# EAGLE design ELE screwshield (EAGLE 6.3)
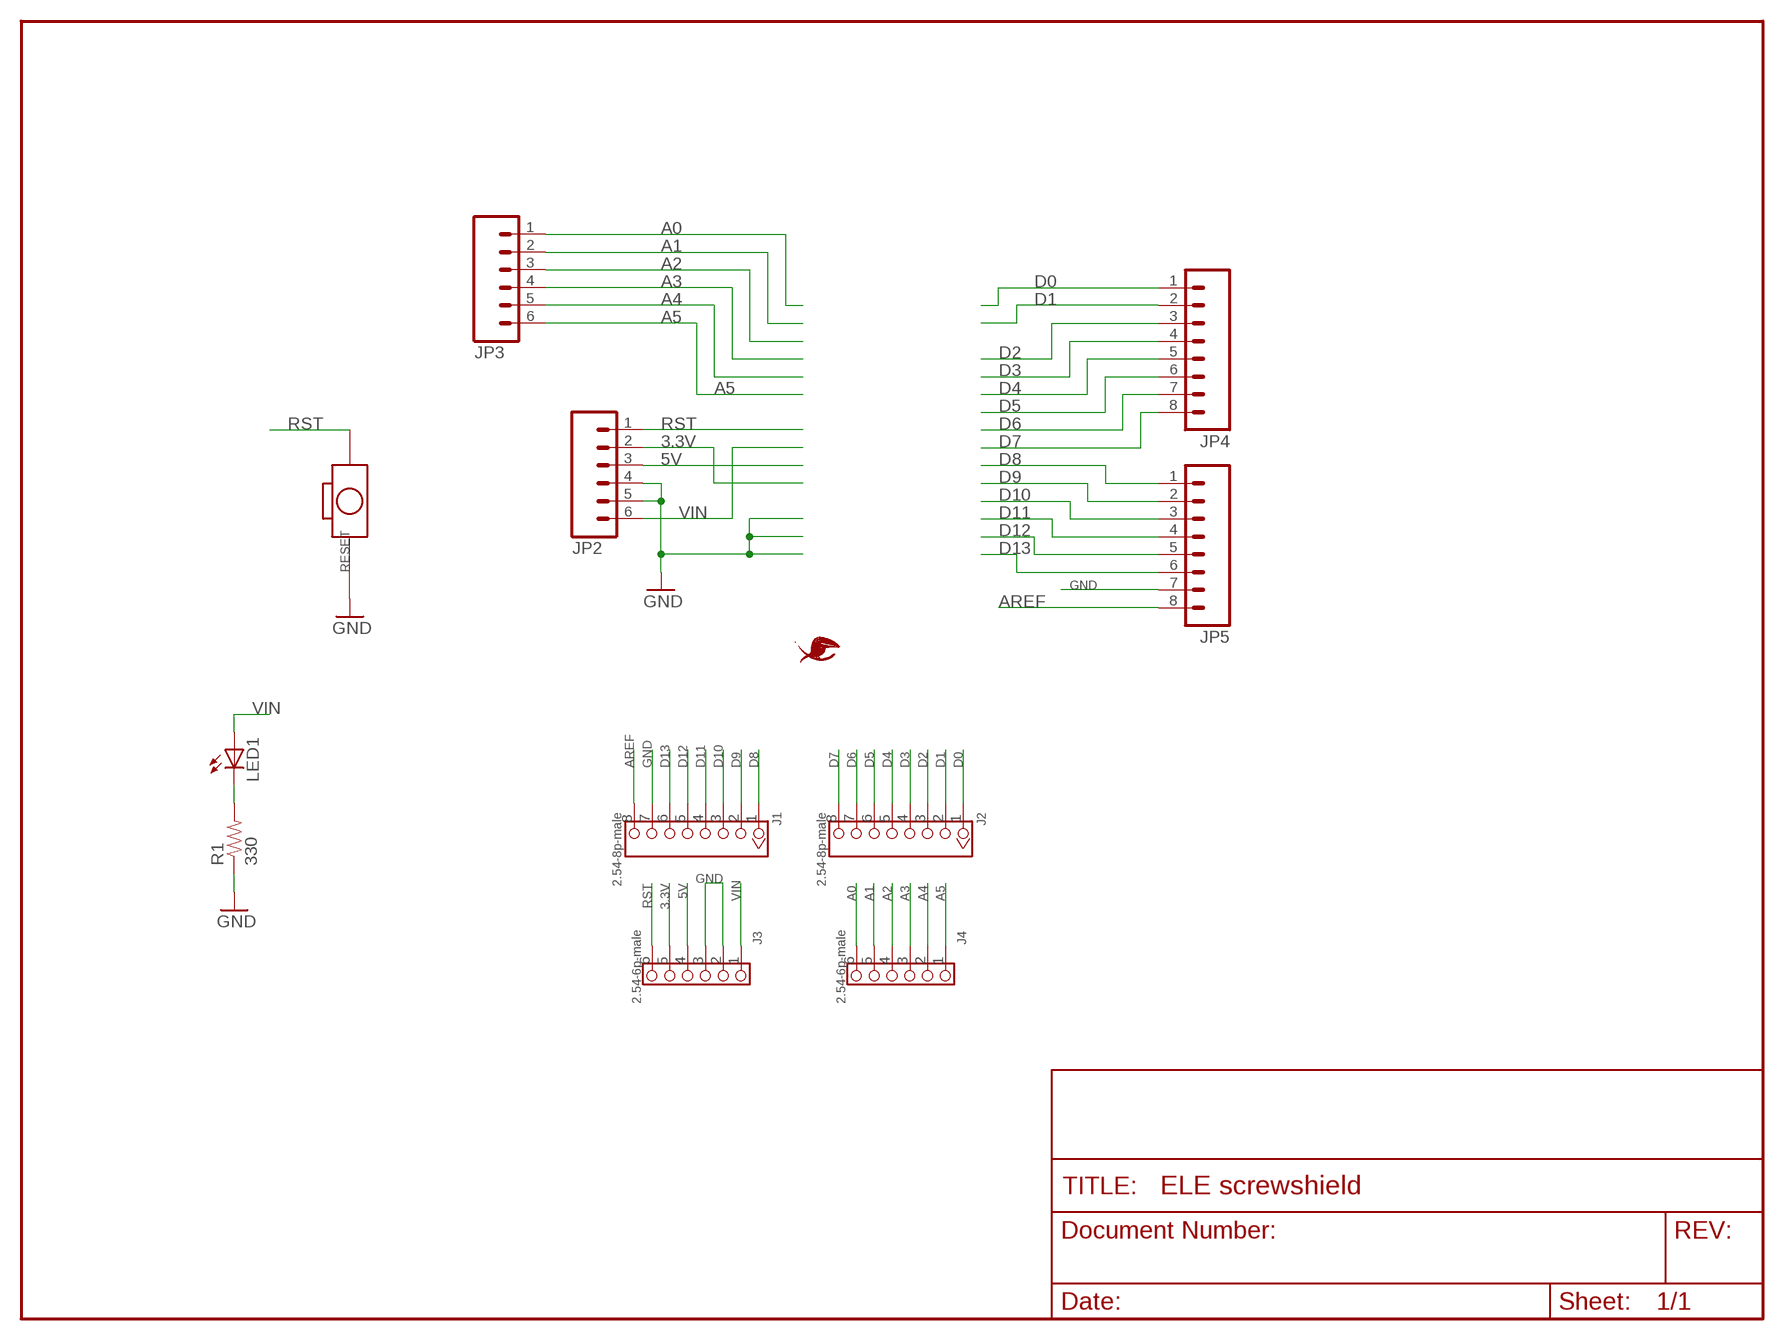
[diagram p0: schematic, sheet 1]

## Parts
J1  2.54-8p-male  HEADER-8P-2.54  [8P-2.54]
J2  2.54-8p-male  HEADER-8P-2.54  [8P-2.54]
J3  2.54-6p-male  HEADER-6P-65/35MIL  [6P-2.54-65/35MIL]
J4  2.54-6p-male  HEADER-6P-65/35MIL  [6P-2.54-65/35MIL]
JP2  M063.5MM-6  [SCREWTERMINAL-3.5MM-6]
JP3  M063.5MM-6  [SCREWTERMINAL-3.5MM-6]
JP4  M083.5MM-8  [SCREWTERMINAL-3.5MM-8]
JP5  M083.5MM-8  [SCREWTERMINAL-3.5MM-8]
LED1  LED5MM  [LED5MM]
R1  330  RESISTORPTH1  [AXIAL-0.3]
RESET  BOTTON-2P-90D  [2P-7.62X3.56-90D]
U$2  ELECROW3  [ELECROW3]

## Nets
3.3V: J3.5 JP2.2
5V: J3.4 JP2.3
A0: J4.6 JP3.1
A1: J4.5 JP3.2
A2: J4.4 JP3.3
A3: J4.3 JP3.4
A4: J4.2 JP3.5
A5: J4.1 JP3.6
AREF: J1.8 JP5.8
D0: J2.1 JP4.1
D1: J2.2 JP4.2
D2: J2.3 JP4.3
D3: J2.4 JP4.4
D4: J2.5 JP4.5
D5: J2.6 JP4.6
D6: J2.7 JP4.7
D7: J2.8 JP4.8
D8: J1.1 JP5.1
D9: J1.2 JP5.2
D10: J1.3 JP5.3
D11: J1.4 JP5.4
D12: J1.5 JP5.5
D13: J1.6 JP5.6
GND: J1.7 J3.2 J3.3 JP2.4 JP2.5 JP5.7 R1.P$1 RESET.P$1
N$6: LED1.K(C) R1.P$2
RST: J3.6 JP2.1 RESET.P$2
VIN: J3.1 JP2.6 LED1.A

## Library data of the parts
J1 J2 = Connector:HEADER-8P
J3 J4 = Connector:HEADER-6P
JP2 JP3 = SparkFun:M06: Header 6 Standard 6-pin 0.1" header. Use with straight break away headers (SKU : PRT-00116), right angle break away headers (PRT-00553), swiss pins (PRT-00743), machine pins (PRT-00117), and female headers (PRT-00115). Molex polarized connector foot print use with SKU : PRT-08094 with associated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
JP4 JP5 = SparkFun:M08: Header 8 Standard 8-pin 0.1" header. Use with straight break away headers (SKU : PRT-00116), right angle break away headers (PRT-00553), swiss pins (PRT-00743), machine pins (PRT-00117), and female headers (PRT-00115).
LED1 = SparkFun:LED: LEDs
R1 = SparkFun:RESISTOR: Resistor
RESET = Discrete:BOTTON-2P
U$2 = ELECROW:ELECROW3

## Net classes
0 default: width 0.152 mm, drill 0.305 mm, clearance 0.152 mm

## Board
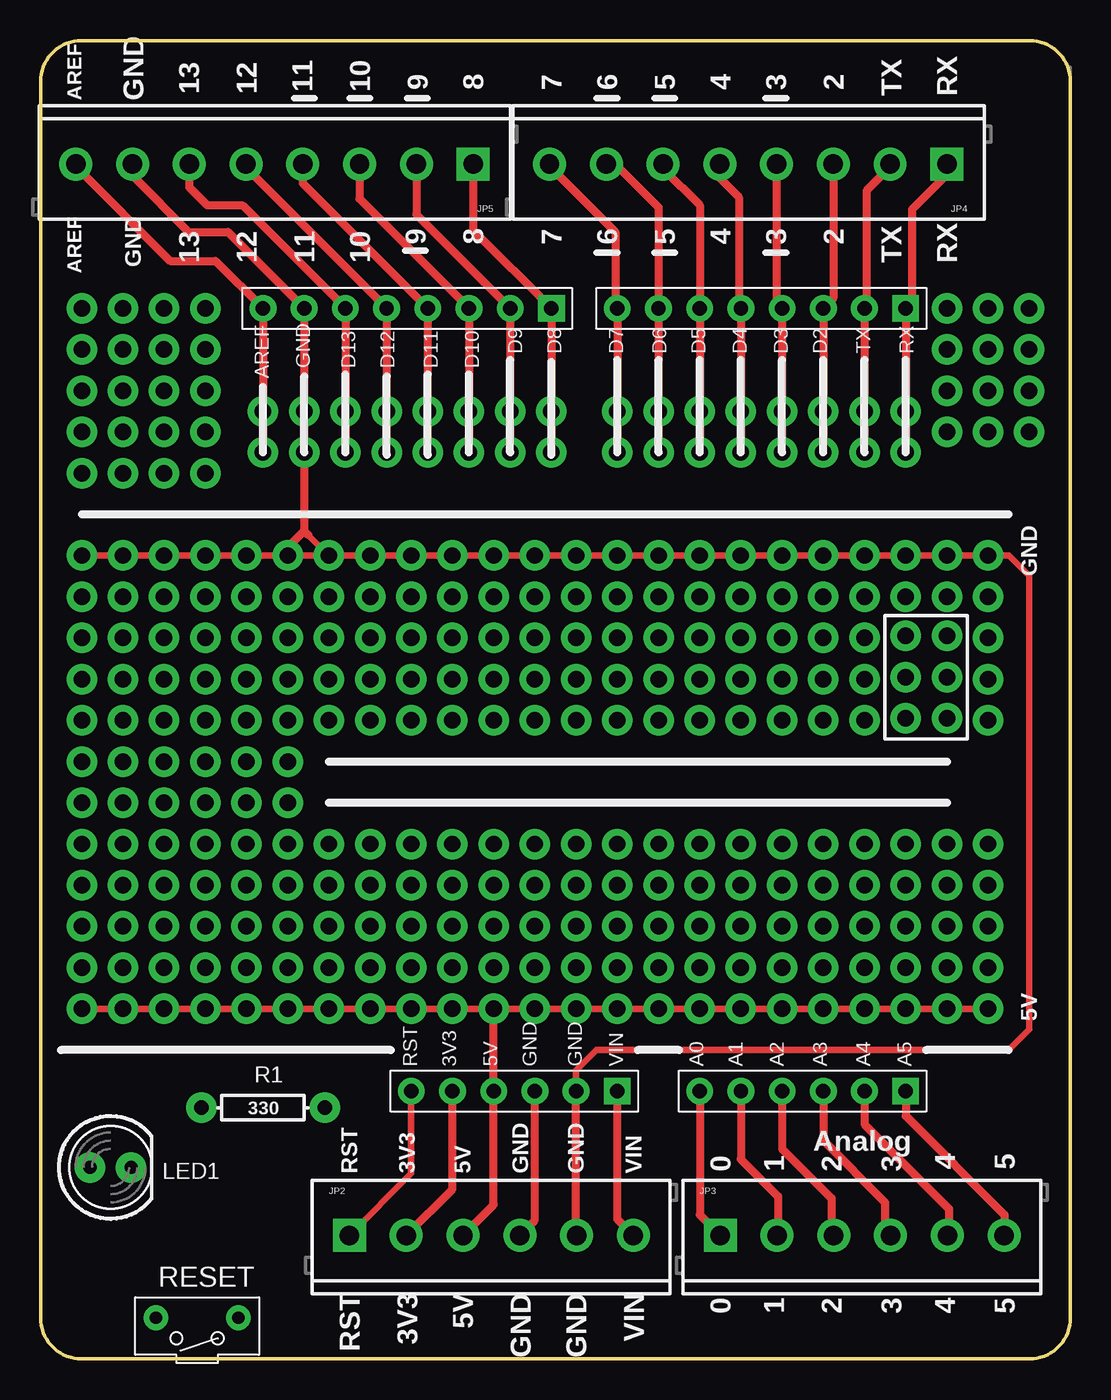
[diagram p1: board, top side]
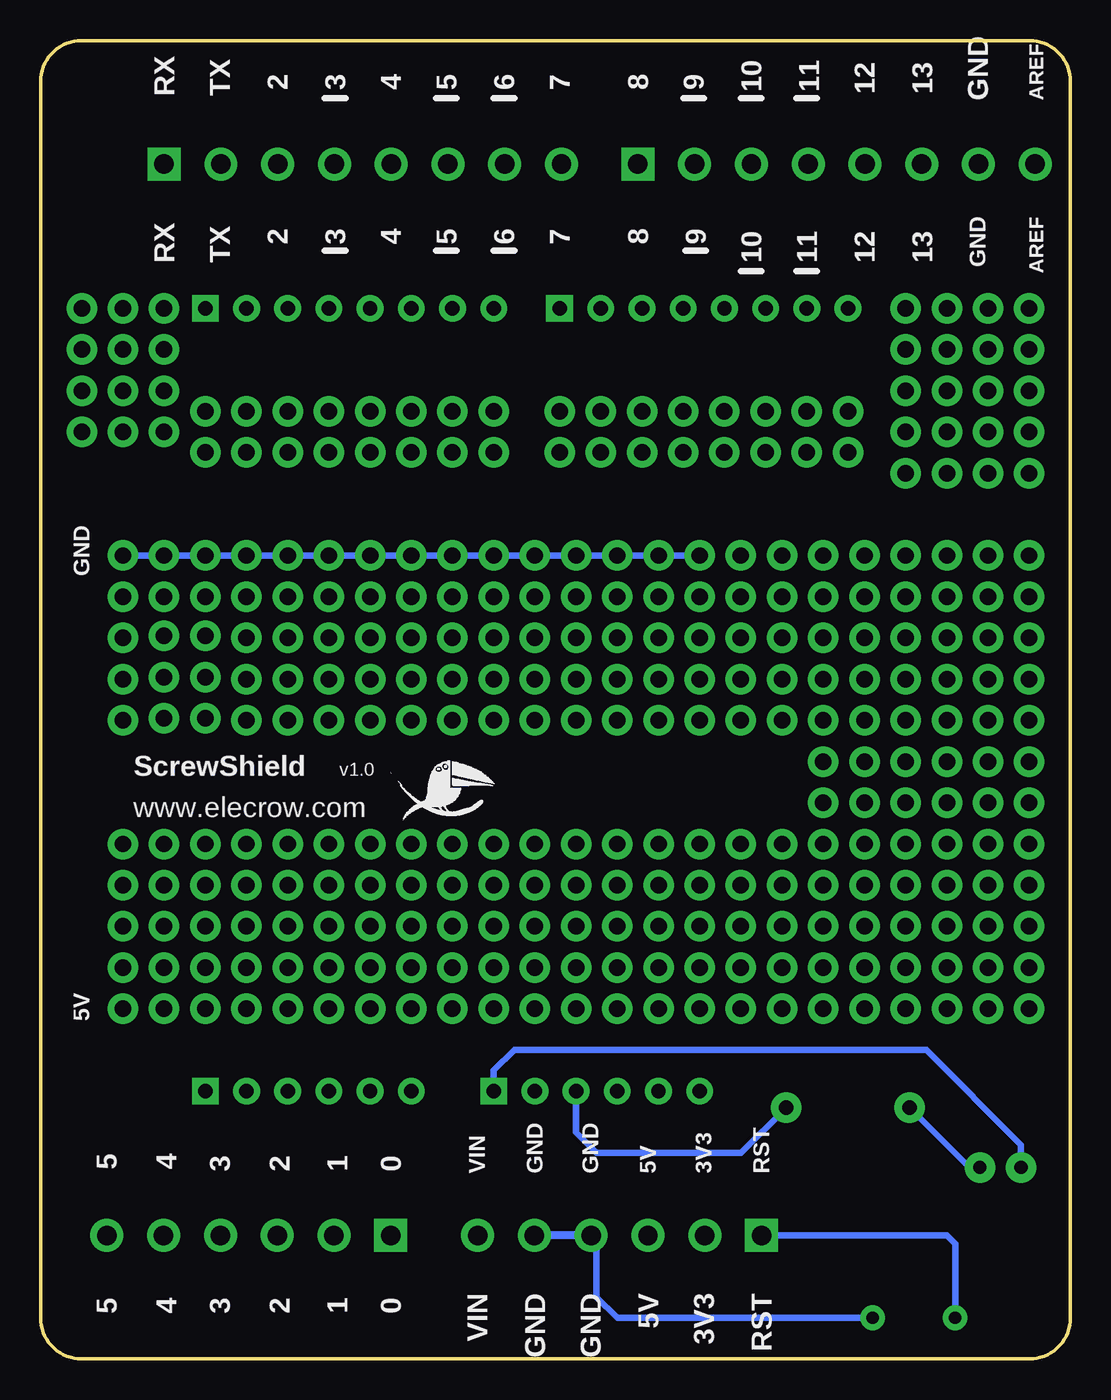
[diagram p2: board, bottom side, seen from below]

Size 63.5 x 81.28 mm. Coordinates in mm from the lower left corner, seen from the top.
Outline: 2.54,0 60.96,0 arc90 63.5,2.54 63.5,78.74 arc90 60.96,81.28 2.54,81.28 arc90 0,78.74 0,2.54 arc90 2.54,0
Copper layers (1*16): Top 0.035mm / dielectric 1.5mm / Bottom 0.035mm
Design rules "SparkFun": minimum track width 8mil, minimum drill 20mil, track to track 8mil, track to pad 8mil, pad to pad 8mil, via to via 8mil, smd to smd 8mil, copper to edge 9mil, drill to drill 8mil, minimum pad ring 12mil, minimum via ring 10mil, stop-mask expansion 4mil, vias tented up to drill 20mil, thermal gap 10mil

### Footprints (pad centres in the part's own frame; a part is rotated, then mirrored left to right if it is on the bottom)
8P-2.54 = drill 0.889 pad 1.651 square: 1 0,8.89 | drill 0.889 pad 1.651: 2 0,6.35; 3 0,3.81; 4 0,1.27; 5 0,-1.27; 6 0,-3.81; 7 0,-6.35; 8 0,-8.89
6P-2.54-65/35MIL = drill 0.889 pad 1.651 square: 1 0,6.35 | drill 0.889 pad 1.651: 2 0,3.81; 3 0,1.27; 4 0,-1.27; 5 0,-3.81; 6 0,-6.35
SCREWTERMINAL-3.5MM-6 = drill 1.2 pad 2.032 square: 1 0,0 | drill 1.2 pad 2.032: 2 3.5,0; 3 7,0; 4 10.5,0; 5 14,0; 6 17.5,0
SCREWTERMINAL-3.5MM-8 = drill 1.2 pad 2.032 square: 1 0,0 | drill 1.2 pad 2.032: 2 3.5,0; 3 7,0; 4 10.5,0; 5 14,0; 6 17.5,0; 7 21,0; 8 24.5,0
LED5MM = drill 0.813 pad 1.88: A -1.27,0; K 1.27,0
AXIAL-0.3 = drill 0.9 pad 1.88: P$1 -3.81,0; P$2 3.81,0
2P-7.62X3.56-90D = drill 0.762 pad 1.524: P$1 0,2.54; P$2 0,-2.54

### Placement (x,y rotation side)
J1  22.61,64.77 270 top
J2  44.45,64.77 270 top
J3  29.21,16.51 270 top
J4  46.99,16.51 270 top
JP2  19.05,7.62 0 top
JP3  41.91,7.62 0 top
JP4  55.88,73.66 180 top
JP5  26.67,73.66 180 top
LED1  4.32,11.81 0 top
R1  13.72,15.49 180 top
RESET  9.65,2.54 270 top
U$2  42.04,32.13 0 bottom

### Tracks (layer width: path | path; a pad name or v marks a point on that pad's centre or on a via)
3.3V
  Top 0.508: J3.5 25.4,10.47 JP2.2
5V  (via drill 1.02 pad 1.88)
  Top 0.406: v2.54,21.59 v5.08,21.59 v7.62,21.59 v10.16,21.59 v12.7,21.59 v15.24,21.59 v17.78,21.59 v20.32,21.59 v22.86,21.59 v25.4,21.59 v27.94,21.59 v30.48,21.59 v33.02,21.59 v35.56,21.59 v38.1,21.59 v40.64,21.59 v43.18,21.59 v45.72,21.59 v48.26,21.59 v50.8,21.59 v53.34,21.59 v55.88,21.59 v58.42,21.59
  Top 0.508: JP2.3 27.94,9.51 J3.4 v27.94,21.59
A0
  Top 0.508: J4.6 40.64,8.89 JP3.1
A1
  Top 0.508: J4.5 43.18,12.32 45.47,10.03 45.47,7.68 JP3.2
A2
  Top 0.508: J4.4 45.72,12.95 48.77,9.91 48.77,7.76 JP3.3
A3
  Top 0.508: J4.3 48.26,13.46 52.07,9.65 52.07,7.96 JP3.4
A4
  Top 0.508: J4.2 50.8,14.48 56.01,9.27 56.01,7.72 JP3.5
A5
  Top 0.508: J4.1 53.34,14.99 59.44,8.89 59.44,7.65 JP3.6
AREF  (via drill 1.02 pad 1.88)
  Top 0.508: JP5.8 2.17,73.52 8,67.69 10.79,67.69 J1.8 v13.72,58.42 v13.72,55.88
D0  (via drill 1.02 pad 1.88)
  Top 0.508: JP4.1 55.88,73.03 53.72,70.87 53.72,65.15 J2.1 v53.34,58.42 v53.34,55.88
D1  (via drill 1.02 pad 1.88)
  Top 0.508: JP4.2 52.38,73.46 50.93,72.01 50.93,64.9 J2.2 v50.8,58.42 v50.8,55.88
D2  (via drill 1.02 pad 1.88)
  Top 0.508: JP4.3 48.88,65.39 J2.3 v48.26,58.42 v48.26,55.88
D3  (via drill 1.02 pad 1.88)
  Top 0.508: JP4.4 45.38,65.11 J2.4 v45.72,58.42 v45.72,55.88
D4  (via drill 1.02 pad 1.88)
  Top 0.508: JP4.5 41.88,72.8 43.05,71.63 43.05,64.9 J2.5 v43.18,58.42 v43.18,55.88
D5  (via drill 1.02 pad 1.88)
  Top 0.508: JP4.6 38.38,73.38 40.64,71.12 J2.6 v40.64,58.42 v40.64,55.88
D6  (via drill 1.02 pad 1.88)
  Top 0.254: 38.1,64.26 J2.7
  Top 0.508: JP4.7 35.43,73.66 38.1,70.99 38.1,64.26 v38.1,58.42 v38.1,55.88
D7  (via drill 1.02 pad 1.88)
  Top 0.508: JP4.8 31.38,73.52 35.43,69.47 35.43,64.9 J2.8 v35.56,58.42 v35.56,55.88
D8  (via drill 1.02 pad 1.88)
  Top 0.508: JP5.1 26.67,69.6 J1.1 v31.5,58.42 v31.5,55.88
D9  (via drill 1.02 pad 1.88)
  Top 0.508: JP5.2 23.17,70.56 J1.2 v28.96,58.42 v28.96,55.88
D10  (via drill 1.02 pad 1.88)
  Top 0.508: JP5.3 19.67,71.52 J1.3 v26.42,58.42 v26.42,55.88
D11  (via drill 1.02 pad 1.88)
  Top 0.508: JP5.4 16.17,72.48 J1.4 v23.88,58.42 v23.88,55.88
D12  (via drill 1.02 pad 1.88)
  Top 0.508: JP5.5 12.67,73.44 J1.5 v21.34,58.42 v21.34,55.88
D13  (via drill 1.02 pad 1.88)
  Top 0.508: JP5.6 9.17,72.24 10.29,71.12 12.45,71.12 J1.6 v18.8,58.42 v18.8,55.88
GND  (via drill 1.02 pad 1.88)
  Top 0.406: J3.2 33.02,17.78 34.29,19.05 59.69,19.05 60.96,20.32 60.96,48.26 59.69,49.53 v58.42,49.53 v20.32,49.53 v17.78,49.53 | v17.78,49.53 v15.24,49.53 v12.7,49.53 v10.16,49.53 v7.62,49.53 v5.08,49.53 v2.54,49.53 | v17.78,49.53 16.51,50.8
  Top 0.508: J3.2 33.02,7.65 JP2.5 | J3.3 30.48,8.55 JP2.4 | JP5.7 5.67,72.94 9.14,69.47 11.56,69.47 J1.7 v16.26,58.42 v16.26,55.88 16.26,51.05 | 16.26,51.05 16.51,50.8 | v15.24,49.53 15.24,50.04 16.26,51.05
  Bottom 0.254: JP2.5 33.02,7.59
  Bottom 0.406: JP2.4 29.21,7.28 29.21,3.81 27.94,2.54 RESET.P$1 | R1.P$1 20.32,12.7 29.21,12.7 30.48,13.97 J3.3 | v22.86,49.53 v25.4,49.53 v27.94,49.53 v30.48,49.53 v33.02,49.53 v35.56,49.53 v38.1,49.53 v40.64,49.53 v43.18,49.53 v45.72,49.53 v48.26,49.53 v50.8,49.53 v53.34,49.53 v55.88,49.53 v58.42,49.53
  Bottom 0.508: JP2.4 JP2.5
N$2  (via drill 1.02 pad 1.88)
  other vias: 25.4,29.21
N$3  (via drill 1.02 pad 1.88)
  other vias: 27.94,29.21
N$4  (via drill 1.02 pad 1.88)
  other vias: 22.86,24.13
N$5  (via drill 1.02 pad 1.88)
  other vias: 10.16,64.77
N$6
  Bottom 0.406: LED1.K 6.22,11.81 R1.P$2
N$9  (via drill 1.02 pad 1.88)
  other vias: 2.54,24.13
N$11  (via drill 1.02 pad 1.88)
  other vias: 5.08,24.13
N$12  (via drill 1.02 pad 1.88)
  other vias: 5.08,59.69
N$13  (via drill 1.02 pad 1.88)
  other vias: 5.08,57.15
N$14  (via drill 1.02 pad 1.88)
  other vias: 7.62,57.15
N$15  (via drill 1.02 pad 1.88)
  other vias: 7.62,59.69
N$16  (via drill 1.02 pad 1.88)
  other vias: 10.16,59.69
N$17  (via drill 1.02 pad 1.88)
  other vias: 10.16,57.15
N$18  (via drill 1.02 pad 1.88)
  other vias: 7.62,24.13
N$19  (via drill 1.02 pad 1.88)
  other vias: 10.16,24.13
N$20  (via drill 1.02 pad 1.88)
  other vias: 12.7,24.13
N$22  (via drill 1.02 pad 1.88)
  other vias: 15.24,24.13
N$24  (via drill 1.02 pad 1.88)
  other vias: 17.78,24.13
N$25  (via drill 1.02 pad 1.88)
  other vias: 20.32,24.13
N$33  (via drill 1.02 pad 1.88)
  other vias: 45.72,24.13
N$34  (via drill 1.02 pad 1.88)
  other vias: 48.26,24.13
N$35  (via drill 1.02 pad 1.88)
  other vias: 50.8,24.13
N$38  (via drill 1.02 pad 1.88)
  other vias: 53.34,24.13
N$39  (via drill 1.02 pad 1.88)
  other vias: 55.88,24.13
N$40  (via drill 1.02 pad 1.88)
  other vias: 58.42,24.13
N$43  (via drill 1.02 pad 1.88)
  other vias: 55.88,59.69
N$44  (via drill 1.02 pad 1.88)
  other vias: 58.42,59.69
N$45  (via drill 1.02 pad 1.88)
  other vias: 60.96,59.69
N$46  (via drill 1.02 pad 1.88)
  other vias: 43.18,24.13
N$49  (via drill 1.02 pad 1.88)
  other vias: 55.88,57.15
N$51  (via drill 1.02 pad 1.88)
  other vias: 58.42,57.15
N$52  (via drill 1.02 pad 1.88)
  other vias: 60.96,57.15
N$53  (via drill 1.02 pad 1.88)
  other vias: 30.48,29.21
N$73  (via drill 1.02 pad 1.88)
  other vias: 33.02,29.21
N$74  (via drill 1.02 pad 1.88)
  other vias: 35.56,29.21
N$75  (via drill 1.02 pad 1.88)
  other vias: 38.1,29.21
N$76  (via drill 1.02 pad 1.88)
  other vias: 40.64,29.21
N$77  (via drill 1.02 pad 1.88)
  other vias: 22.86,29.21
N$78  (via drill 1.02 pad 1.88)
  other vias: 2.54,29.21
N$79  (via drill 1.02 pad 1.88)
  other vias: 2.54,26.67
N$80  (via drill 1.02 pad 1.88)
  other vias: 5.08,29.21
N$81  (via drill 1.02 pad 1.88)
  other vias: 7.62,29.21
N$82  (via drill 1.02 pad 1.88)
  other vias: 10.16,29.21
N$83  (via drill 1.02 pad 1.88)
  other vias: 12.7,29.21
N$84  (via drill 1.02 pad 1.88)
  other vias: 15.24,29.21
N$85  (via drill 1.02 pad 1.88)
  other vias: 17.78,29.21
N$86  (via drill 1.02 pad 1.88)
  other vias: 20.32,29.21
N$87  (via drill 1.02 pad 1.88)
  other vias: 5.08,26.67
N$88  (via drill 1.02 pad 1.88)
  other vias: 7.62,26.67
N$89  (via drill 1.02 pad 1.88)
  other vias: 10.16,26.67
N$90  (via drill 1.02 pad 1.88)
  other vias: 12.7,26.67
N$91  (via drill 1.02 pad 1.88)
  other vias: 15.24,26.67
N$92  (via drill 1.02 pad 1.88)
  other vias: 17.78,26.67
N$93  (via drill 1.02 pad 1.88)
  other vias: 20.32,26.67
N$94  (via drill 1.02 pad 1.88)
  other vias: 25.4,26.67
N$95  (via drill 1.02 pad 1.88)
  other vias: 27.94,26.67
N$96  (via drill 1.02 pad 1.88)
  other vias: 30.48,26.67
N$97  (via drill 1.02 pad 1.88)
  other vias: 33.02,26.67
N$98  (via drill 1.02 pad 1.88)
  other vias: 35.56,26.67
N$99  (via drill 1.02 pad 1.88)
  other vias: 38.1,26.67
N$100  (via drill 1.02 pad 1.88)
  other vias: 40.64,26.67
N$101  (via drill 1.02 pad 1.88)
  other vias: 22.86,26.67
N$102  (via drill 1.02 pad 1.88)
  other vias: 45.72,29.21
N$103  (via drill 1.02 pad 1.88)
  other vias: 48.26,29.21
N$104  (via drill 1.02 pad 1.88)
  other vias: 50.8,29.21
N$105  (via drill 1.02 pad 1.88)
  other vias: 53.34,29.21
N$106  (via drill 1.02 pad 1.88)
  other vias: 55.88,29.21
N$107  (via drill 1.02 pad 1.88)
  other vias: 58.42,29.21
N$108  (via drill 1.02 pad 1.88)
  other vias: 43.18,29.21
N$109  (via drill 1.02 pad 1.88)
  other vias: 2.54,41.91
N$110  (via drill 1.02 pad 1.88)
  other vias: 2.54,39.37
N$111  (via drill 1.02 pad 1.88)
  other vias: 5.08,41.91
N$112  (via drill 1.02 pad 1.88)
  other vias: 7.62,41.91
N$113  (via drill 1.02 pad 1.88)
  other vias: 10.16,41.91
N$114  (via drill 1.02 pad 1.88)
  other vias: 12.7,41.91
N$115  (via drill 1.02 pad 1.88)
  other vias: 15.24,41.91
N$116  (via drill 1.02 pad 1.88)
  other vias: 5.08,39.37
N$117  (via drill 1.02 pad 1.88)
  other vias: 7.62,39.37
N$118  (via drill 1.02 pad 1.88)
  other vias: 10.16,39.37
N$119  (via drill 1.02 pad 1.88)
  other vias: 12.7,39.37
N$120  (via drill 1.02 pad 1.88)
  other vias: 15.24,39.37
N$121  (via drill 1.02 pad 1.88)
  other vias: 2.54,46.99
N$122  (via drill 1.02 pad 1.88)
  other vias: 2.54,44.45
N$123  (via drill 1.02 pad 1.88)
  other vias: 5.08,46.99
N$124  (via drill 1.02 pad 1.88)
  other vias: 7.62,46.99
N$125  (via drill 1.02 pad 1.88)
  other vias: 10.16,46.99
N$126  (via drill 1.02 pad 1.88)
  other vias: 12.7,46.99
N$127  (via drill 1.02 pad 1.88)
  other vias: 15.24,46.99
N$128  (via drill 1.02 pad 1.88)
  other vias: 5.08,44.45
N$129  (via drill 1.02 pad 1.88)
  other vias: 45.72,26.67
N$130  (via drill 1.02 pad 1.88)
  other vias: 7.62,44.45
N$131  (via drill 1.02 pad 1.88)
  other vias: 10.16,44.45
N$132  (via drill 1.02 pad 1.88)
  other vias: 12.7,44.45
N$133  (via drill 1.02 pad 1.88)
  other vias: 15.24,44.45
N$140  (via drill 1.02 pad 1.88)
  other vias: 2.54,36.83
N$141  (via drill 1.02 pad 1.88)
  other vias: 2.54,34.29
N$142  (via drill 1.02 pad 1.88)
  other vias: 5.08,36.83
N$143  (via drill 1.02 pad 1.88)
  other vias: 7.62,36.83
N$144  (via drill 1.02 pad 1.88)
  other vias: 10.16,36.83
N$145  (via drill 1.02 pad 1.88)
  other vias: 12.7,36.83
N$146  (via drill 1.02 pad 1.88)
  other vias: 15.24,36.83
N$147  (via drill 1.02 pad 1.88)
  other vias: 5.08,34.29
N$148  (via drill 1.02 pad 1.88)
  other vias: 7.62,34.29
N$149  (via drill 1.02 pad 1.88)
  other vias: 10.16,34.29
N$150  (via drill 1.02 pad 1.88)
  other vias: 48.26,26.67
N$151  (via drill 1.02 pad 1.88)
  other vias: 50.8,26.67
N$152  (via drill 1.02 pad 1.88)
  other vias: 53.34,26.67
N$153  (via drill 1.02 pad 1.88)
  other vias: 55.88,26.67
N$154  (via drill 1.02 pad 1.88)
  other vias: 58.42,26.67
N$155  (via drill 1.02 pad 1.88)
  other vias: 43.18,26.67
N$156  (via drill 1.02 pad 1.88)
  other vias: 25.4,31.75
N$157  (via drill 1.02 pad 1.88)
  other vias: 27.94,31.75
N$158  (via drill 1.02 pad 1.88)
  other vias: 30.48,31.75
N$159  (via drill 1.02 pad 1.88)
  other vias: 33.02,31.75
N$160  (via drill 1.02 pad 1.88)
  other vias: 35.56,31.75
N$161  (via drill 1.02 pad 1.88)
  other vias: 38.1,31.75
N$162  (via drill 1.02 pad 1.88)
  other vias: 40.64,31.75
N$163  (via drill 1.02 pad 1.88)
  other vias: 22.86,31.75
N$164  (via drill 1.02 pad 1.88)
  other vias: 2.54,31.75
N$165  (via drill 1.02 pad 1.88)
  other vias: 5.08,31.75
N$166  (via drill 1.02 pad 1.88)
  other vias: 7.62,31.75
N$167  (via drill 1.02 pad 1.88)
  other vias: 10.16,31.75
N$168  (via drill 1.02 pad 1.88)
  other vias: 12.7,31.75
N$169  (via drill 1.02 pad 1.88)
  other vias: 15.24,31.75
N$170  (via drill 1.02 pad 1.88)
  other vias: 17.78,31.75
N$171  (via drill 1.02 pad 1.88)
  other vias: 20.32,31.75
N$172  (via drill 1.02 pad 1.88)
  other vias: 45.72,31.75
N$173  (via drill 1.02 pad 1.88)
  other vias: 48.26,31.75
N$174  (via drill 1.02 pad 1.88)
  other vias: 50.8,31.75
N$175  (via drill 1.02 pad 1.88)
  other vias: 53.34,31.75
N$176  (via drill 1.02 pad 1.88)
  other vias: 55.88,31.75
N$177  (via drill 1.02 pad 1.88)
  other vias: 58.42,31.75
N$178  (via drill 1.02 pad 1.88)
  other vias: 43.18,31.75
N$179  (via drill 1.02 pad 1.88)
  other vias: 12.7,34.29
N$180  (via drill 1.02 pad 1.88)
  other vias: 15.24,34.29
N$194  (via drill 1.02 pad 1.88)
  other vias: 17.78,39.37
N$195  (via drill 1.02 pad 1.88)
  other vias: 20.32,39.37
N$196  (via drill 1.02 pad 1.88)
  other vias: 22.86,39.37
N$197  (via drill 1.02 pad 1.88)
  other vias: 25.4,39.37
N$198  (via drill 1.02 pad 1.88)
  other vias: 27.94,39.37
N$199  (via drill 1.02 pad 1.88)
  other vias: 30.48,39.37
N$200  (via drill 1.02 pad 1.88)
  other vias: 33.02,39.37
N$201  (via drill 1.02 pad 1.88)
  other vias: 35.56,39.37
N$202  (via drill 1.02 pad 1.88)
  other vias: 38.1,39.37
N$203  (via drill 1.02 pad 1.88)
  other vias: 40.64,39.37
N$204  (via drill 1.02 pad 1.88)
  other vias: 43.18,39.37
N$205  (via drill 1.02 pad 1.88)
  other vias: 45.72,39.37
N$206  (via drill 1.02 pad 1.88)
  other vias: 48.26,39.37
N$207  (via drill 1.02 pad 1.88)
  other vias: 50.8,39.37
N$208  (via drill 1.02 pad 1.88)
  other vias: 53.34,39.5
N$209  (via drill 1.02 pad 1.88)
  other vias: 55.88,39.5
N$210  (via drill 1.02 pad 1.88)
  other vias: 58.42,39.37
N$221  (via drill 1.02 pad 1.88)
  other vias: 17.78,41.91
N$222  (via drill 1.02 pad 1.88)
  other vias: 20.32,41.91
N$223  (via drill 1.02 pad 1.88)
  other vias: 22.86,41.91
N$224  (via drill 1.02 pad 1.88)
  other vias: 25.4,41.91
N$225  (via drill 1.02 pad 1.88)
  other vias: 27.94,41.91
N$226  (via drill 1.02 pad 1.88)
  other vias: 30.48,41.91
N$227  (via drill 1.02 pad 1.88)
  other vias: 33.02,41.91
N$228  (via drill 1.02 pad 1.88)
  other vias: 35.56,41.91
N$229  (via drill 1.02 pad 1.88)
  other vias: 38.1,41.91
N$230  (via drill 1.02 pad 1.88)
  other vias: 40.64,41.91
N$231  (via drill 1.02 pad 1.88)
  other vias: 43.18,41.91
N$232  (via drill 1.02 pad 1.88)
  other vias: 45.72,41.91
N$233  (via drill 1.02 pad 1.88)
  other vias: 48.26,41.91
N$234  (via drill 1.02 pad 1.88)
  other vias: 50.8,41.91
N$235  (via drill 1.02 pad 1.88)
  other vias: 53.34,42.04
N$236  (via drill 1.02 pad 1.88)
  other vias: 55.88,42.04
N$237  (via drill 1.02 pad 1.88)
  other vias: 58.42,41.91
N$248  (via drill 1.02 pad 1.88)
  other vias: 17.78,44.45
N$249  (via drill 1.02 pad 1.88)
  other vias: 20.32,44.45
N$250  (via drill 1.02 pad 1.88)
  other vias: 22.86,44.45
N$251  (via drill 1.02 pad 1.88)
  other vias: 25.4,44.45
N$252  (via drill 1.02 pad 1.88)
  other vias: 27.94,44.45
N$253  (via drill 1.02 pad 1.88)
  other vias: 30.48,44.45
N$254  (via drill 1.02 pad 1.88)
  other vias: 33.02,44.45
N$255  (via drill 1.02 pad 1.88)
  other vias: 35.56,44.45
N$256  (via drill 1.02 pad 1.88)
  other vias: 38.1,44.45
N$257  (via drill 1.02 pad 1.88)
  other vias: 40.64,44.45
N$258  (via drill 1.02 pad 1.88)
  other vias: 43.18,44.45
N$259  (via drill 1.02 pad 1.88)
  other vias: 45.72,44.45
N$260  (via drill 1.02 pad 1.88)
  other vias: 48.26,44.45
N$261  (via drill 1.02 pad 1.88)
  other vias: 50.8,44.45
N$262  (via drill 1.02 pad 1.88)
  other vias: 53.34,44.58
N$263  (via drill 1.02 pad 1.88)
  other vias: 55.88,44.58
N$264  (via drill 1.02 pad 1.88)
  other vias: 58.42,44.45
N$275  (via drill 1.02 pad 1.88)
  other vias: 17.78,46.99
N$276  (via drill 1.02 pad 1.88)
  other vias: 20.32,46.99
N$277  (via drill 1.02 pad 1.88)
  other vias: 22.86,46.99
N$278  (via drill 1.02 pad 1.88)
  other vias: 25.4,46.99
N$279  (via drill 1.02 pad 1.88)
  other vias: 27.94,46.99
N$280  (via drill 1.02 pad 1.88)
  other vias: 30.48,46.99
N$281  (via drill 1.02 pad 1.88)
  other vias: 33.02,46.99
N$282  (via drill 1.02 pad 1.88)
  other vias: 35.56,46.99
N$283  (via drill 1.02 pad 1.88)
  other vias: 38.1,46.99
N$284  (via drill 1.02 pad 1.88)
  other vias: 40.64,46.99
N$285  (via drill 1.02 pad 1.88)
  other vias: 43.18,46.99
N$286  (via drill 1.02 pad 1.88)
  other vias: 45.72,46.99
N$287  (via drill 1.02 pad 1.88)
  other vias: 48.26,46.99
N$288  (via drill 1.02 pad 1.88)
  other vias: 50.8,46.99
N$289  (via drill 1.02 pad 1.88)
  other vias: 53.34,46.99
N$290  (via drill 1.02 pad 1.88)
  other vias: 55.88,46.99
N$291  (via drill 1.02 pad 1.88)
  other vias: 58.42,46.99
N$350  (via drill 1.02 pad 1.88)
  other vias: 2.54,54.61
N$351  (via drill 1.02 pad 1.88)
  other vias: 5.08,54.61
N$352  (via drill 1.02 pad 1.88)
  other vias: 7.62,54.61
N$353  (via drill 1.02 pad 1.88)
  other vias: 10.16,54.61
N$377  (via drill 1.02 pad 1.88)
  other vias: 2.54,57.15
N$404  (via drill 1.02 pad 1.88)
  other vias: 2.54,59.69
N$439  (via drill 1.02 pad 1.88)
  other vias: 25.4,24.13
N$440  (via drill 1.02 pad 1.88)
  other vias: 27.94,24.13
N$441  (via drill 1.02 pad 1.88)
  other vias: 30.48,24.13
N$442  (via drill 1.02 pad 1.88)
  other vias: 33.02,24.13
N$443  (via drill 1.02 pad 1.88)
  other vias: 35.56,24.13
N$444  (via drill 1.02 pad 1.88)
  other vias: 38.1,24.13
N$445  (via drill 1.02 pad 1.88)
  other vias: 40.64,24.13
N$447  (via drill 1.02 pad 1.88)
  other vias: 2.54,62.23
N$448  (via drill 1.02 pad 1.88)
  other vias: 5.08,62.23
N$449  (via drill 1.02 pad 1.88)
  other vias: 7.62,62.23
N$455  (via drill 1.02 pad 1.88)
  other vias: 10.16,62.23
N$457  (via drill 1.02 pad 1.88)
  other vias: 2.54,64.77
N$458  (via drill 1.02 pad 1.88)
  other vias: 5.08,64.77
N$459  (via drill 1.02 pad 1.88)
  other vias: 7.62,64.77
N$478  (via drill 1.02 pad 1.88)
  other vias: 55.88,62.23
N$479  (via drill 1.02 pad 1.88)
  other vias: 58.42,62.23
N$480  (via drill 1.02 pad 1.88)
  other vias: 60.96,62.23
N$488  (via drill 1.02 pad 1.88)
  other vias: 55.88,64.77
N$489  (via drill 1.02 pad 1.88)
  other vias: 58.42,64.77
N$490  (via drill 1.02 pad 1.88)
  other vias: 60.96,64.77
RST
  Top 0.406: J3.6 22.86,11.43 JP2.1
  Bottom 0.406: JP2.1 7.62,7.62 7.11,7.11 RESET.P$2
VIN
  Top 0.508: J3.1 35.56,8.61 JP2.6
  Bottom 0.406: LED1.A 3.05,13.21 8.89,19.05 34.29,19.05 35.56,17.78 J3.1

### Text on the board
tPlace: AREF | GND | 13 | 12 | 11 | 10 | 9 | 8 | 7 | 6 | 5 | 4 | 3 | 2 | TX | RX | 9 | 8 | 7 | 6 | 5 | 4 | 3 | 2 | 13 | 12 | 11 | 10 | TX | RX | AREF | GND | D9 | D8 | D7 | D6 | D5 | D4 | D3 | D2 | TX | RX | GND | D13 | D12 | D11 | D10 | AREF | GND | 5V | RST | 3V3 | 5V | GND | GND | VIN | A0 | A1 | A2 | A3 | A4 | A5 | Analog | 0 | 1 | 2 | 3 | 4 | 5 | RST | 3V3 | 5V | GND | GND | VIN | RST | 3V3 | 5V | GND | GND | VIN | 0 | 1 | 2 | 3 | 4 | 5
bPlace: AREF | GND | 13 | 12 | 11 | 10 | 9 | 8 | 7 | 6 | 5 | 4 | 3 | 2 | TX | RX | 9 | 8 | 7 | 6 | 5 | 4 | 3 | 2 | 13 | 12 | 11 | 10 | TX | RX | AREF | GND | GND | v1.0 | ScrewShield | www.elecrow.com | 5V | 0 | 1 | 2 | 3 | 4 | 5 | RST | 3V3 | 5V | GND | GND | VIN | RST | 3V3 | 5V | GND | GND | VIN | 0 | 1 | 2 | 3 | 4 | 5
